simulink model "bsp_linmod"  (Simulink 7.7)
settings: Solver=ode45  StartTime=0.0  StopTime=0.5  RelTol=1e-3

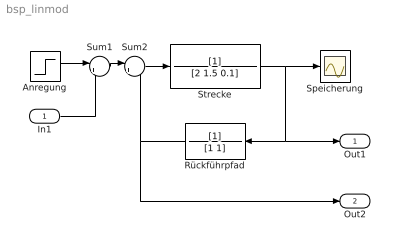
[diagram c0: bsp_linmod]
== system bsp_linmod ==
  In1 : Inport
  Anregung : Step  SampleTime=0
  Rückführpfad : TransferFcn  Denominator=[1 1]
  Speicherung : Scope
  Strecke : TransferFcn  Denominator=[2 1.5 0.1]
  Sum1 : Sum  Inputs=|++
  Sum2 : Sum  Inputs=|+-
  Out1 : Outport
  Out2 : Outport  Port=2
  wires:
  Sum2/1 -> Strecke/1
  Rückführpfad/1 -> Sum2/2, Out2/1
  Strecke/1 -> Rückführpfad/1, Out1/1, Speicherung/1
  Anregung/1 -> Sum1/1
  Sum1/1 -> Sum2/1
  In1/1 -> Sum1/2
